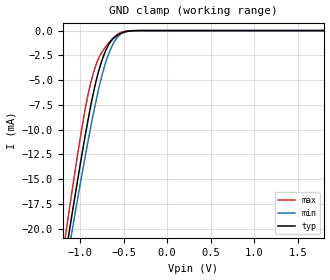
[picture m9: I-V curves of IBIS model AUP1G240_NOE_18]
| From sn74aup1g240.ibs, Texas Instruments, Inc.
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[Model]   AUP1G240_NOE_18
Model_type  Input
Vinl=0.6825
Vinh=1.0725
| variable   typ   min   max
C_comp   1.66pF   1.45pF   1.92pF
[Temperature Range]   40   100   -40
| Ambient temperature   25   85   -40
[Voltage range]   1.8   1.65   1.95
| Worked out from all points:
|   GND clamp passes 1 mA (typ) near -0.64 V on its own axis
[GND Clamp]
| AUP1G240_NOE_18
|   Voltage   I(typ)   I(min)   I(max)
-3.6V     -171.6mA   -163.5mA   -181.1mA
-1.16V    -22.22mA   -23.69mA   -20.18mA
-1.135V   -20.83mA   -22.39mA   -18.68mA
-1.11V    -19.45mA   -21.09mA   -17.19mA
-1.09V    -18.36mA   -20.06mA   -16.01mA
-960mV    -11.5mA    -13.57mA   -8.799mA
-850mV    -6.372mA   -8.471mA   -4.359mA
-780mV    -3.86mA    -5.615mA   -2.659mA
-710mV    -2.096mA   -3.313mA   -1.67mA
-625mV    -855.5uA   -1.409mA   -788.9uA
-540mV    -313.2uA   -390uA     -224.9uA
1.8V      83.14pA    451.3pA    18.98pA
